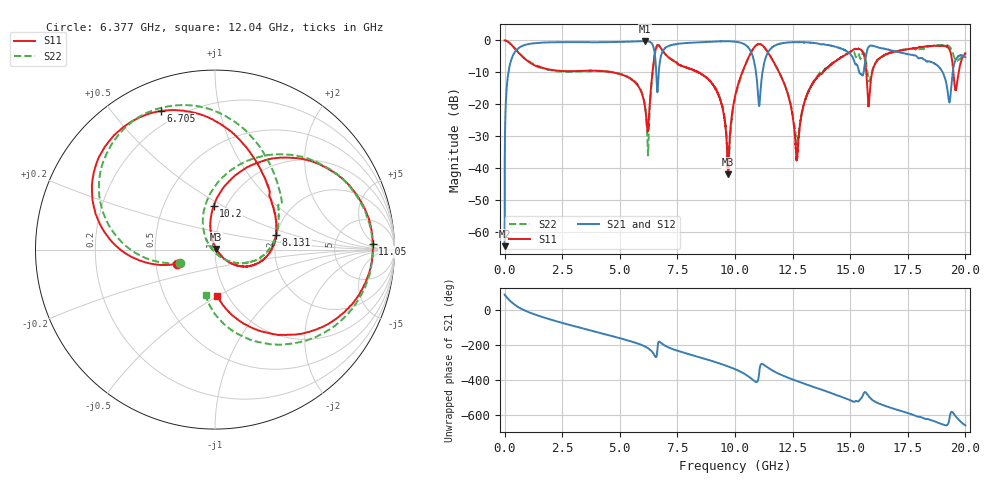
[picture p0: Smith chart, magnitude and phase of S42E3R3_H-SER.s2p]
!{S42E3R3}
!Johanson Technology Inc.
!www.johansontechnology.com
!Test Board Conditions:
!Substrate Type  RO4350B
!Substrate Thickness  50 mil
!Substrate Dk  3.66
!TL Type: GCPW
!TL Trace Width  60 mil
!TL Gap  10 mil
!Electrode orientation  Horizontal
!DUT TOPOLOGY	SERIES
!Mounting Pad LxW  14x55 mil
! Created Wed Nov 25 21:43:10 2020
# khz S ma R 50
! 2 Port Network Data from SP1.SP block
! freq  magS11  angS11  magS21  angS21  magS12  angS12  magS22  angS22
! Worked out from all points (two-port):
!   20001 points, 300 kHz to 20 GHz, reference 50 ohm
!   highest |S21| = -0.20 dB at 6.082 GHz (marker M1); lowest = -64.5 dB at 300 kHz (marker M2)
!   |S21| within 3 dB of the highest: 488.6 MHz to 6.497 GHz (6.008 GHz wide, 172 % of centre); 6.877 GHz to 10.67 GHz (3.792 GHz wide, 43.2 % of centre)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
!   lowest |S11| = -42.0 dB at 9.702 GHz (marker M3), VSWR 1.02, Z = 50.7 + j0.397 ohm
!   |S11| at or under -10 dB: 4.701 GHz to 6.418 GHz (1.717 GHz wide, 30.9 % of centre); 8.417 GHz to 10.31 GHz (1.896 GHz wide, 20.2 % of centre); 11.92 GHz to 13.81 GHz (1.898 GHz wide, 14.8 % of centre)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
!   |S22| runs from -39.7 to 0.0 dB; largest |S21 - S12| = 0.021
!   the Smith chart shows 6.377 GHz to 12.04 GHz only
!   S11 on the Smith chart (normalised r, x): 6.377 GHz: 0.65, -0.11; 6.705 GHz: 0.14, +0.67; 8.131 GHz: 1.98, +0.38; 10.2 GHz: 0.88, +0.45; 11.05 GHz: 15, +4; 12.04 GHz: 0.90, -0.49
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300  1 -0.3  0.0005984 91.5  0.000613 89.7  0.9993 -0.2
122300  0.9695 -18.3  0.2391 71.3  0.2401 71.3  0.9694 -18.4
408300  0.7719 -54.2  0.6283 36.2  0.6292 36.2  0.7746 -54.2
1333300  0.4023 -114.3  0.9069 -24.0  0.9053 -24.0  0.4137 -114.5
3334300  0.3333 165.7  0.9405 -101.1  0.9397 -101.1  0.3275 171.4
6082300  0.0964 81.9  0.9769 154.2  0.9755 154.2  0.1011 64.9
6377300  0.2249 -159.4  0.9121 126.9  0.9138 126.9  0.2106 -159.5
6667300  0.85 121.6  0.2351 175.0  0.2356 174.6  0.8506 114.7
6705300  0.8294 111.4  0.3656 -179.0  0.3659 -179.4  0.8287 104.0
8131300  0.3504 13.7  0.9208 103.9  0.9174 104.1  0.3479 13.0
9244300  0.1505 -36.0  0.9639 59.6  0.9677 59.6  0.1557 -28.6
9702300  0.007977 29.4  0.9717 38.6  0.9722 38.5  0.01217 -103.7
1.00003e7  0.1324 101.5  0.9576 23.0  0.9572 23.0  0.1227 120.8
1.02023e7  0.2442 91.7  0.9299 10.9  0.9308 10.9  0.2323 104.9
1.10543e7  0.8796 2.0  0.09453 8.6  0.09505 9.4  0.8781 -0.8
1.20373e7  0.2554 -87.6  0.9023 -11.4  0.9046 -11.7  0.2574 -101.7
1.26843e7  0.01408 -33.5  0.9412 -45.0  0.9415 -45.2  0.02569 -58.6
1.33343e7  0.1994 21.4  0.9183 -75.8  0.9192 -75.7  0.2046 -2.8
1.66673e7  0.6282 -101.1  0.7161 165.4  0.7002 165.3  0.6227 -111.3
1.92873e7  0.7423 125.5  0.1123 84.7  0.1137 84.6  0.8131 136.1
1.95893e7  0.1693 149.7  0.508 110.0  0.5128 109.6  0.4921 126.7
2e7  0.6204 165.5  0.5454 60.3  0.5466 61.1  0.6314 130.3
